[IBIS Ver]  4.0
[File Name]  lpc2478fet.ibs
[File Rev]  1.0
[Date]  Mon Dec 18 10:34:29 2006
[Source]  Package model from Ansoft Q3D Extractor 7.1.1
[Notes]   IO models Rev 0.20 IBIS Model Design Automation Generation
[Copyright]  NXP Semiconductors 2006,2007. All rights reserved.
|   lpc2478FET (208 TFBGA package) IBIS Model
[Disclaimer]
| NXP Semiconductors warrants and represents that the IBIS models
| identified herein are owned by NXP Semiconductors (NXP).  The
| models provided are not warranted as fully representing all of the
| operating characteristics and specifications of the semiconductor
| products to which the models relate.  Moreover, unless there is a
| signed, written agreement to the contrary, these models are furnished
| on an "as is" basis without support or warranty of any kind, either
| expressed or implied, regarding the use thereof, and NXP
| specifically disclaims all implied warranties of merchantability and
| fitness of the models for any purpose.
| NXP does not assume any liability arising out of the application
| or use of these IBIS models including infringement of patents and
| copyrights, nor does NXP convey any license under its patents and
| copyrights or the rights of others.
| NXP provides IBIS models as a service to our customers.  You and
| your company shall not distribute, convey, sell, or give these models
| to anyone else without receiving prior written permission from
| NXP.
[Define Package Model]  TFBGA208
[Manufacturer]  NXP Semiconductors
[OEM]  NXP Semiconductors
[Description]  TFBGA208
|   A full package IBIS model
|   Bondwires, bga balls, vias and all interconnect are included.
|Sim freq: 100 MHz
|Date: 12/18/06
[Number Of Pins]  182
[Pin Numbers]
F4   | 10 = dbgen
U1   | 58 = dmb
M2   | 41 = nreset
U15   | 102 = port0<0>
T15   | 106 = port0<10>
R14   | 108 = port0<11>
R1   | 47 = port0<12>
R2   | 51 = port0<13>
T7   | 75 = port0<14>
J16   | 140 = port0<15>
J14   | 142 = port0<16>
K17   | 138 = port0<17>
K15   | 136 = port0<18>
L17   | 134 = port0<19>
T14   | 104 = port0<1>
M17   | 131 = port0<20>
M16   | 129 = port0<21>
N17   | 126 = port0<22>
H1   | 19 = port0<23>
G2   | 17 = port0<24>
F1   | 15 = port0<25>
E1   | 13 = port0<26>
T1   | 56 = port0<27>
U4   | 67 = port0<29>
C4   | 219 = port0<2>
R6   | 68 = port0<30>
T2   | 57 = port0<31>
D6   | 221 = port0<3>
B12   | 183 = port0<4>
C12   | 181 = port0<5>
D13   | 179 = port0<6>
C13   | 177 = port0<7>
A15   | 175 = port0<8>
C14   | 173 = port0<9>
A3   | 213 = port1<0>
C8   | 203 = port1<10>
A14   | 178 = port1<11>
A16   | 172 = port1<12>
D16   | 161 = port1<13>
A7   | 201 = port1<14>
A8   | 199 = port1<15>
D10   | 197 = port1<16>
A9   | 195 = port1<17>
P7   | 72 = port1<18>
U6   | 74 = port1<19>
B5   | 211 = port1<1>
U7   | 76 = port1<20>
R8   | 78 = port1<21>
U8   | 80 = port1<22>
P9   | 82 = port1<23>
T9   | 84 = port1<24>
T10   | 86 = port1<25>
R10   | 88 = port1<26>
T12   | 96 = port1<27>
T13   | 98 = port1<28>
U14   | 100 = port1<29>
D9   | 202 = port1<2>
P2   | 48 = port1<30>
P1   | 46 = port1<31>
A10   | 194 = port1<3>
A5   | 209 = port1<4>
A17   | 171 = port1<5>
B11   | 186 = port1<6>
C7   | 207 = port1<8>
A6   | 205 = port1<9>
B17   | 169 = port2<0>
N15   | 119 = port2<10>
T17   | 117 = port2<11>
N14   | 115 = port2<12>
T16   | 110 = port2<13>
R12   | 99 = port2<14>
P13   | 107 = port2<15>
R11   | 95 = port2<16>
R13   | 103 = port2<17>
U3   | 65 = port2<18>
R7   | 73 = port2<19>
E14   | 167 = port2<1>
T8   | 79 = port2<20>
U11   | 87 = port2<21>
U12   | 92 = port2<22>
U5   | 70 = port2<23>
P5   | 59 = port2<24>
R4   | 60 = port2<25>
T4   | 63 = port2<26>
P3   | 53 = port2<27>
P4   | 55 = port2<28>
N3   | 49 = port2<29>
D15   | 165 = port2<2>
L4   | 35 = port2<30>
N2   | 45 = port2<31>
E16   | 158 = port2<3>
D17   | 156 = port2<4>
F16   | 152 = port2<5>
E17   | 150 = port2<6>
G16   | 148 = port2<7>
H15   | 146 = port2<8>
H16   | 144 = port2<9>
B4   | 214 = port3<0>
B2   | 222 = port3<10>
D5   | 225 = port3<11>
D4   | 1 = port3<12>
C1   | 7 = port3<13>
H2   | 22 = port3<14>
M1   | 31 = port3<15>
F17   | 149 = port3<16>
F15   | 157 = port3<17>
C15   | 166 = port3<18>
B14   | 176 = port3<19>
B3   | 218 = port3<1>
A13   | 182 = port3<20>
C10   | 192 = port3<21>
C6   | 212 = port3<22>
T6   | 71 = port3<23>
R5   | 64 = port3<24>
U2   | 62 = port3<25>
T3   | 61 = port3<26>
A1   | 220 = port3<27>
D2   | 5 = port3<28>
F3   | 12 = port3<29>
B1   | 224 = port3<2>
H3   | 20 = port3<30>
J3   | 27 = port3<31>
E4   | 3 = port3<3>
F2   | 14 = port3<4>
G1   | 18 = port3<5>
J1   | 24 = port3<6>
L1   | 30 = port3<7>
D8   | 208 = port3<8>
C5   | 216 = port3<9>
U9   | 81 = port4<0>
G17   | 147 = port4<10>
F14   | 159 = port4<11>
C16   | 163 = port4<12>
B16   | 170 = port4<13>
B15   | 174 = port4<14>
A11   | 189 = port4<15>
U17   | 109 = port4<16>
P14   | 112 = port4<17>
P15   | 114 = port4<18>
P16   | 120 = port4<19>
U10   | 85 = port4<1>
R17   | 118 = port4<20>
M15   | 125 = port4<21>
K14   | 135 = port4<22>
J15   | 141 = port4<23>
B8   | 200 = port4<24>
B9   | 196 = port4<25>
L15   | 130 = port4<26>
G15   | 151 = port4<27>
C11   | 185 = port4<28>
B10   | 193 = port4<29>
T11   | 89 = port4<2>
B7   | 204 = port4<30>
A4   | 210 = port4<31>
U16   | 105 = port4<3>
R15   | 111 = port4<4>
R16   | 116 = port4<5>
M14   | 123 = port4<6>
L16   | 132 = port4<7>
J17   | 139 = port4<8>
H17   | 143 = port4<9>
K3   | 32 = rstoutn
N1   | 43 = rtc_alarm_lp
C3   | 223 = rtck
K2   | 40 = rtcx1
L2   | 42 = rtcx2
E2   | 11 = tck
C2   | 4 = tdi
D3   | 2 = tdo
E3   | 6 = tms
D1   | 8 = trst_n
D14   | 168 = port1<7>
R3   | 54 = port0<28>
H4   | 28 = v3
G4   | 21 = v3a
P11   | 93 = v3e_1
D11   | 190 = v3e_2
M3   | 44 = vbat
K1   | 25 = vrefp
J2   | 23 = vssa_adc
M4   | 50 = x1
N4   | 52 = x2
[Model Data]
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[End Model Data]
[End Package Model]
|| [End]
[Component]   lpc2478FET
[Manufacturer]  NXP
[Package]
|   typ   min   max
R_pkg   0   0   0  |Values included in package model
L_pkg   0   0   0  |Values included in package model
C_pkg   0   0   0  |Values included in package model
[Package Model]  TFBGA208
| (Pin and IO model definitions)
| IMPORTANT NOTES:
| The LPC2478 GPIO pins, excluding the I2C and USB, have programmable input
| configurations. For this reason, three models are supplied for those basic
| padcells. Each model is identified by a unique suffix code at the end of
| the modelname:
| _p=plain input, _pd=pulldown enabled, _pu=pullup enabled
| The model_name for each of the GPIO pins in the [Pin] table below reflects
| the default state of that pin on power up (input with pullup enabled).
| The user may modify the model_name for a specific P#.# pin if that pin's
| input configuration is programmed differently from the default in the
| actual application. However, the model_names for all other pins are
| non-configurable and should not be altered.
| All GPIO padcells have 5ns slew rate control when operated as outputs,
| unless otherwise noted.
[Pin]   signal_name   model_name   | comments
D4   P3.12   bpts5ptpht5v_pu   |
D3   TDO   bpts5ptpht5v_p   | 3-state output only
E4   P3.3   bpts5ptpht5v_pu   |
C2   TDI   bpts5ptpht5v_pu   | In only
D2   P3.28   bpts5ptpht5v_pu   |
E3   TMS   bpts5ptpht5v_pu   | In only
C1   P3.13   bpts5ptpht5v_pu   |
D1   TRST_N   bpts5ptpht5v_pu   | In only
F4   DBGEN   bpts5ptpht5v_pu   | In only
E2   TCK   bpts5ptpht5v_p   | In only
F3   P3.29   bpts5ptpht5v_pu   |
E1   P0.26   bpats5thpept5v_pu |
F2   P3.4   bpts5ptpht5v_pu   |
F1   P0.25   bpats5thpept5v_pu |
G2   P0.24   bpats5thpept5v_pu |
G1   P3.5   bpts5ptpht5v_pu   |
H1   P0.23   bpats5thpept5v_pu |
H3   P3.30   bpts5ptpht5v_pu   |
G4   VddA   POWER
H2   P3.14   bpts5ptpht5v_pu   |
J2   VssA   GND
J1   P3.6   bpts5ptpht5v_pu   |
K1   VrefA   POWER
J3   P3.31   bpts5ptpht5v_pu   |
H4   Vddcore   NC   | check???
L1   P3.7   bpts5ptpht5v_pu   |
M1   P3.15   bpts5ptpht5v_pu   |
K3   RSTOUTN   bpts5ptpht5v_pu   | Output only
L4   P2.30   bpts5ptpht5v_pu   |
K2   RTCX1   NC
M2   NRESET   bpts5ptpht5v_pu   | In only
L2   RTCX2   NC
N1   ALARM   bptpcph1v8   | Output only, 1.8V, no slew
M3   VBAT   POWER
N2   P2.31   bpts5ptpht5v_pu   |
P1   P1.31   bpats5thpept5v_pu |
R1   P0.12   bpats5thpept5v_pu |
P2   P1.30   bpats5thpept5v_pu |
N3   P2.29   bpts5ptpht5v_pu   |
M4   X1   NC
R2   P0.13   bpats5thpept5v_pu |
N4   X2   NC
P3   P2.27   bpts5ptpht5v_pu   |
R3   P0.28   iic3m4sdat5v_400k | I2C padcell
P4   P2.28   bpts5ptpht5v_pu   |
T1   P0.27   iic3m4sdat5v_400k | I2C padcell
T2   P0.31   usb11f1_iop_hs   | USB padcell
U1   DMB   usb11f1_iom_hs   | USB padcell
P5   P2.24   bpts5ptpht5v_pu   |
R4   P2.25   bpts5ptpht5v_pu   |
T3   P3.26   bpts5ptpht5v_pu   |
U2   P3.25   bpts5ptpht5v_pu   |
T4   P2.26   bpts5ptpht5v_pu   |
R5   P3.24   bpts5ptpht5v_pu   |
U3   P2.18   bpts5ptpht5v_pu   |
U4   P0.29   usb11f1_iop_hs   | USB padcell
R6   P0.30   usb11f1_iom_hs   | USB padcell
U5   P2.23   bpts5ptpht5v_pu   |
T6   P3.23   bpts5ptpht5v_pu   |
P7   P1.18   bpts5ptpht5v_pu   |
R7   P2.19   bpts5ptpht5v_pu   |
U6   P1.19   bpts5ptpht5v_pu   |
T7   P0.14   bpts5ptpht5v_pu   |
U7   P1.20   bpts5ptpht5v_pu   |
R8   P1.21   bpts5ptpht5v_pu   |
T8   P2.20   bpts5ptpht5v_pu   |
U8   P1.22   bpts5ptpht5v_pu   |
U9   P4.0   bpts5ptpht5v_pu   |
P9   P1.23   bpts5ptpht5v_pu   |
T9   P1.24   bpts5ptpht5v_pu   |
U10   P4.1   bpts5ptpht5v_pu   |
T10   P1.25   bpts5ptpht5v_pu   |
U11   P2.21   bpts5ptpht5v_pu   |
R10   P1.26   bpts5ptpht5v_pu   |
T11   P4.2   bpts5ptpht5v_pu   |
U12   P2.22   bpts5ptpht5v_pu   |
P11   Vdd   POWER
R11   P2.16   bpts5ptpht5v_pu   |
T12   P1.27   bpts5ptpht5v_pu   |
T13   P1.28   bpts5ptpht5v_pu   |
R12   P2.14   bpts5ptpht5v_pu   |
U14   P1.29   bpts5ptpht5v_pu   |
U15   P0.0   bpts5ptpht5v_pu   |
R13   P2.17   bpts5ptpht5v_pu   |
T14   P0.1   bpts5ptpht5v_pu   |
U16   P4.3   bpts5ptpht5v_pu   |
T15   P0.10   bpts5ptpht5v_pu   |
P13   P2.15   bpts5ptpht5v_pu   |
R14   P0.11   bpts5ptpht5v_pu   |
U17   P4.16   bpts5ptpht5v_pu   |
T16   P2.13   bpts5ptpht5v_pu   |
R15   P4.4   bpts5ptpht5v_pu   |
P14   P4.17   bpts5ptpht5v_pu   |
P15   P4.18   bpts5ptpht5v_pu   |
N14   P2.12   bpts5ptpht5v_pu   |
R16   P4.5   bpts5ptpht5v_pu   |
T17   P2.11   bpts5ptpht5v_pu   |
R17   P4.20   bpts5ptpht5v_pu   |
N15   P2.10   bpts5ptpht5v_pu   |
P16   P4.19   bpts5ptpht5v_pu   |
M14   P4.6   bpts5ptpht5v_pu   |
M15   P4.21   bpts5ptpht5v_pu   |
N17   P0.22   bpts5ptpht5v_pu   |
M16   P0.21   bpts5ptpht5v_pu   |
L15   P4.26   bpts5ptpht5v_pu   |
M17   P0.20   bpts5ptpht5v_pu
L16   P4.7   bpts5ptpht5v_pu   |
L17   P0.19   bpts5ptpht5v_pu   |
K14   P4.22   bpts5ptpht5v_pu   |
K15   P0.18   bpts5ptpht5v_pu   |
K17   P0.17   bpts5ptpht5v_pu   |
J17   P4.8   bpts5ptpht5v_pu   |
J16   P0.15   bpts5ptpht5v_pu   |
J15   P4.23   bpts5ptpht5v_pu   |
J14   P0.16   bpts5ptpht5v_pu   |
H17   P4.9   bpts5ptpht5v_pu   |
H16   P2.9   bpts5ptpht5v_pu   |
H15   P2.8   bpts5ptpht5v_pu   |
G17   P4.10   bpts5ptpht5v_pu   |
G16   P2.7   bpts5ptpht5v_pu   |
F17   P3.16   bpts5ptpht5v_pu   |
E17   P2.6   bpts5ptpht5v_pu   |
G15   P4.27   bpts5ptpht5v_pu   |
F16   P2.5   bpts5ptpht5v_pu   |
D17   P2.4   bpts5ptpht5v_pu   |
F15   P3.17   bpts5ptpht5v_pu   |
E16   P2.3   bpts5ptpht5v_pu   |
F14   P4.11   bpts5ptpht5v_pu   |
D16   P1.13   bpts5ptpht5v_pu   |
C16   P4.12   bpts5ptpht5v_pu   |
D15   P2.2   bpts5ptpht5v_pu   |
C15   P3.18   bpts5ptpht5v_pu   |
E14   P2.1   bpts5ptpht5v_pu   |
D14   P1.7   bpts5ptpht5v_pu   |
B17   P2.0   bpts5ptpht5v_pu   |
B16   P4.13   bpts5ptpht5v_pu   |
A17   P1.5   bpts5ptpht5v_pu   |
A16   P1.12   bpts5ptpht5v_pu   |
C14   P0.9   bpts5ptpht5v_pu   |
B15   P4.14   bpts5ptpht5v_pu   |
A15   P0.8   bpts5ptpht5v_pu   |
B14   P3.19   bpts5ptpht5v_pu   |
C13   P0.7   bpts5ptpht5v_pu   |
A14   P1.11   bpts5ptpht5v_pu   |
D13   P0.6   bpts5ptpht5v_pu   |
C12   P0.5   bpts5ptpht5v_pu   |
A13   P3.20   bpts5ptpht5v_pu   |
B12   P0.4   bpts5ptpht5v_pu   |
C11   P4.28   bpts5ptpht5v_pu   |
B11   P1.6   bpts5ptpht5v_pu   |
A11   P4.15   bpts5ptpht5v_pu   |
D11   Vdd   POWER
C10   P3.21   bpts5ptpht5v_pu   |
B10   P4.29   bpts5ptpht5v_pu   |
A10   P1.3   bpts5ptpht5v_pu   |
A9   P1.17   bpts5ptpht5v_pu   |
B9   P4.25   bpts5ptpht5v_pu   |
D10   P1.16   bpts5ptpht5v_pu   |
A8   P1.15   bpts5ptpht5v_pu   |
B8   P4.24   bpts5ptpht5v_pu   |
A7   P1.14   bpts5ptpht5v_pu   |
D9   P1.2   bpts5ptpht5v_pu   |
C8   P1.10   bpts5ptpht5v_pu   |
B7   P4.30   bpts5ptpht5v_pu   |
A6   P1.9   bpts5ptpht5v_pu   |
C7   P1.8   bpts5ptpht5v_pu   |
D8   P3.8   bpts5ptpht5v_pu   |
A5   P1.4   bpts5ptpht5v_pu   |
A4   P4.31   bpts5ptpht5v_pu   |
B5   P1.1   bpts5ptpht5v_pu   |
C6   P3.22   bpts5ptpht5v_pu   |
A3   P1.0   bpts5ptpht5v_pu   |
B4   P3.0   bpts5ptpht5v_pu   |
C5   P3.9   bpts5ptpht5v_pu   |
B3   P3.1   bpts5ptpht5v_pu   |
C4   P0.2   bpts5ptpht5v_pu   |
A1   P3.27   bpts5ptpht5v_pu   |
D6   P0.3   bpts5ptpht5v_pu   |
B2   P3.10   bpts5ptpht5v_pu   |
C3   RTCK   bpts5ptpht5v_pu   |
B1   P3.2   bpts5ptpht5v_pu   |
D5   P3.11   bpts5ptpht5v_pu   |
| Models and submodels in the file (10): bpats5thpept5v_p (I/O), bpats5thpept5v_pd (I/O), bpats5thpept5v_pu (I/O), bpts5ptpht5v_p (I/O), bpts5ptpht5v_pd (I/O), bpts5ptpht5v_pu (I/O), iic3m4sdat5v_400k (I/O_open_drain), usb11f1_iom_hs (I/O), usb11f1_iop_hs (I/O), bptpcph1v8 (Output)
